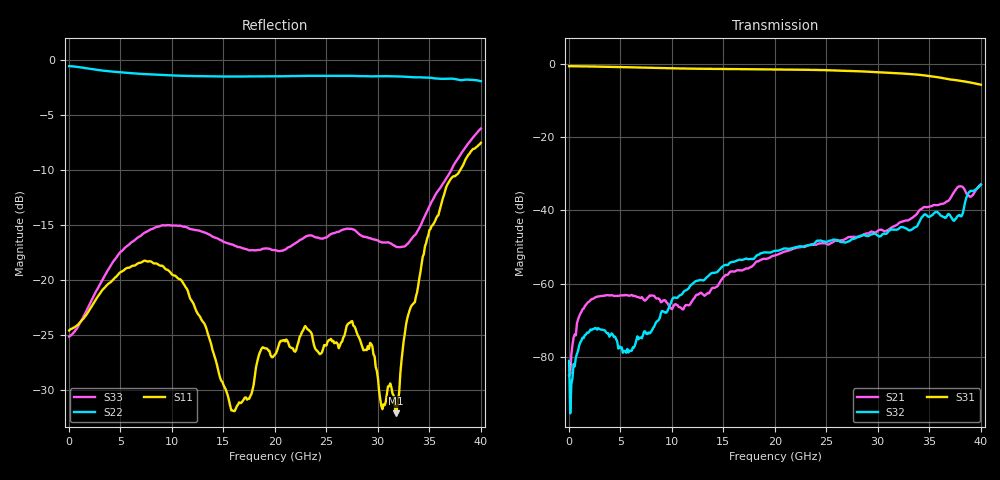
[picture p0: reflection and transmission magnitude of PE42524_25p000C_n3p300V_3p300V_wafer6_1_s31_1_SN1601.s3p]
!Agilent Technologies,N5224A,MY51441010,A.09.90.07
!Agilent N5224A: A.09.90.07
!Date: Wednesday, September 10, 2014 09:35:42
!Correction: S11(Full 3 Port(1,2,3))
!S12(Full 3 Port(1,2,3))
!S13(Full 3 Port(1,2,3))
!S21(Full 3 Port(1,2,3))
!S22(Full 3 Port(1,2,3))
!S23(Full 3 Port(1,2,3))
!S31(Full 3 Port(1,2,3))
!S32(Full 3 Port(1,2,3))
!S33(Full 3 Port(1,2,3))
!S3P File: Measurements: <S11,S12,S13>,
!<S21,S22,S23>,
!<S31,S32,S33>:
# Hz S  dB  R 50
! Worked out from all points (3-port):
!   369 points, 10 MHz to 40.02 GHz, reference 50 ohm
!   strongest paths, dB at 10 MHz, 10.01 GHz, 20.02 GHz, 30.02 GHz, 40.02 GHz:
!     S31: -0.6, -1.2, -1.4, -2.2, -5.6
!     S32: -81.1, -64.4, -51.0, -46.9, -33.0
!     S21: -85.1, -67.0, -52.3, -45.5, -32.9
!   lowest |S11| = -32.1 dB at 31.76 GHz (marker M1), VSWR 1.05, Z = 49.6 + j2.44 ohm
!   |S11| at or under -10 dB: start of sweep to 38 GHz
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1e7  -24.58 -0.7  -85.62 6.8  -0.58 -0.2
     -85.09 -53.2  -0.52 179.9  -85.98 -9.1
     -0.58 -0.2  -81.08 15.9  -25.14 -0.5
2.075775e9  -22.57 -59.0  -64.47 35.7  -0.66 -28.0
            -64.52 35.5  -0.77 162.7  -72.55 12.1
            -0.66 -28.0  -72.54 10.4  -22.05 -69.4
7.512025e9  -18.27 -156.5  -64.32 -0.8  -1.00 -99.6
            -64.32 0.0  -1.25 123.0  -73.73 145.9
            -1.00 -99.7  -73.71 145.0  -15.61 -169.3
1.370935e10  -25.52 102.9  -62.07 21.9  -1.31 -179.7
             -62.06 21.7  -1.45 76.5  -57.39 54.0
             -1.31 -179.8  -57.41 54.2  -15.88 110.8
1.599258e10  -31.91 21.8  -56.70 4.2  -1.36 150.4
             -56.71 4.0  -1.47 58.5  -54.01 14.3
             -1.36 150.3  -54.03 14.1  -16.81 86.5
2.00154e10  -26.78 -96.7  -52.28 -28.6  -1.44 96.7
            -52.30 -28.5  -1.45 25.5  -51.05 -50.6
            -1.44 96.6  -51.03 -50.8  -17.28 46.2
2.6104e10  -25.82 -120.0  -48.28 -94.9  -1.78 12.2
           -48.28 -94.9  -1.41 -27.3  -48.07 -151.7
           -1.78 12.1  -48.07 -151.8  -15.61 -41.6
3.17577e10  -32.12 97.0  -44.14 -145.7  -2.48 -69.6
            -44.12 -145.7  -1.45 -76.4  -45.26 140.1
            -2.47 -69.7  -45.27 140.2  -16.95 -99.1
3.501945e10  -15.44 -10.9  -38.98 173.8  -3.30 -120.0
             -38.97 173.7  -1.57 -105.4  -41.76 105.5
             -3.29 -120.2  -41.77 105.4  -13.29 -111.3
4.00208e10  -7.50 -87.2  -32.88 118.3  -5.65 161.5
            -32.87 118.2  -1.89 -151.2  -32.95 76.2
            -5.64 161.3  -32.96 76.2  -6.20 -170.0
